(* Logix 5000 DataType export EdDSA_INTERNAL; software revision 30.00 *)

TYPE EdDSA_INTERNAL :
STRUCT
   MsgCopy : EdDSA_MSG;
   MsgToBeVerified : EdDSA_MSG;
   MsgLastVerified : EdDSA_MSG;
   MsgInProcessing : EdDSA_MSG;
   MsgToBeSent : EdDSA_MSG;
   VerifyQue : DINT;
   ProcessQue : DINT;
   VerificationInProgress : BOOL;
   VerificationStatus : DINT;
   ProcessingRequired : BOOL;
   ProcessingInProgress : BOOL;
   ProcessingStatus : DINT;
END_STRUCT
END_TYPE

TYPE EdDSA_MSG :
STRUCT
   Status : CONNECTION_STATUS;
   Flags : DINT;
   PubDH : STRING;
   Ke : STRING;
   KsID : LINT;
   KsPrimeID : LINT;
   Counter : LINT;
   Sig_R : STRING;
   Sig_S : STRING;
END_STRUCT
END_TYPE
